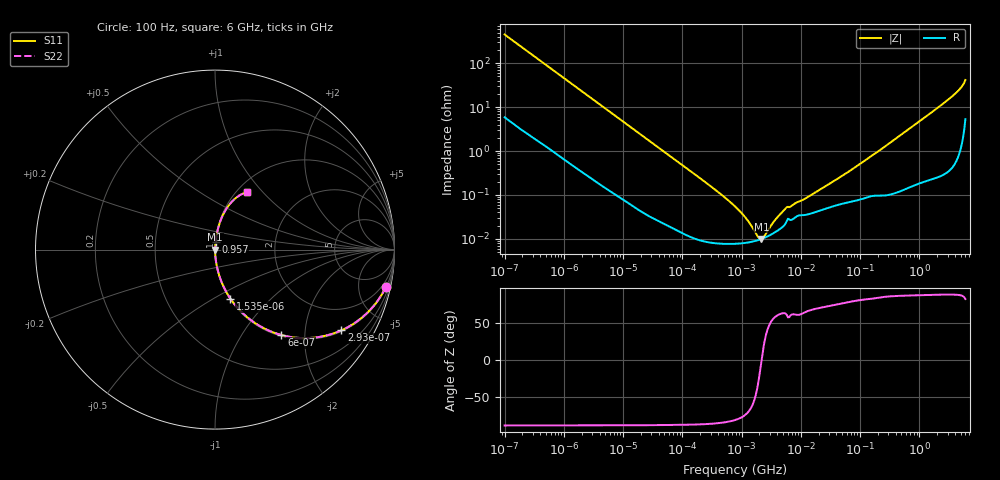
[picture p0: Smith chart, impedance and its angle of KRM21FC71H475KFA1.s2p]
!Murata Part Number: KRM21FC71H475KFA1
!These Parameters are Measured in Series Mode Connection
!Data Generated on Jan 08, 2026
!  o--ll--o
!Port1  Port2
!  o------o
!Operation Temp=25[degC], DC Bias Voltage=0[V]
!Freq. Start=100[Hz] Stop=6[GHz] 401[Steps]
# Hz S RI R 50
!Freq.(Hz) S11(Real) S11(Imag) S21(Real) S21(Imag) S12(Real) S12(Imag) S22(Real) S22(Imag)
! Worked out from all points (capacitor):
!   401 points, 100 Hz to 6 GHz, reference 50 ohm
!   read as one part in series: C = 3.52 uF near 109 Hz
!   lowest |Z| = 9.97 mohm at 2.169 MHz (marker M1)
!   series resonance near 2.178 MHz, so ESL is about 1.5 nH
!   S11 on the Smith chart (normalised r, x): 100 Hz: 1.12, -9.02; 293 Hz: 1.04, -3.11; 600 Hz: 1.02, -1.53; 1.535 kHz: 1.01, -0.60; 957 MHz: 1.00, +0.09; 6 GHz: 1.11, +0.82
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100  0.9507 -0.2102  0.0493 0.2102  0.0493 0.2102  0.9507 -0.2102
179  0.8619 -0.3386  0.1381 0.3386  0.1381 0.3386  0.8619 -0.3386
293  0.7046 -0.4496  0.2954 0.4496  0.2954 0.4496  0.7046 -0.4496
600  0.3702 -0.4759  0.6298 0.4759  0.6298 0.4759  0.3702 -0.4759
938  0.1971 -0.3908  0.8029 0.3908  0.8029 0.3908  0.1971 -0.3908
1535  0.0862 -0.2737  0.9138 0.2737  0.9138 0.2737  0.0862 -0.2737
2008  0.0533 -0.2175  0.9467 0.2175  0.9467 0.2175  0.0533 -0.2175
6728  0.00591 -0.0691  0.9941 0.0691  0.9941 0.0691  0.00591 -0.0691
40335  0.000391 -0.0118  0.9996 0.0118  0.9996 0.0118  0.000391 -0.0118
302498  8.45e-05 -0.00157  0.9999 0.00157  0.9999 0.00157  8.45e-05 -0.00157
774597  7.77e-05 -0.000545  0.9999 0.000545  0.9999 0.000545  7.77e-05 -0.000545
1212075  8.19e-05 -0.000274  0.9999 0.000274  0.9999 0.000274  8.19e-05 -0.000274
1896632  9.37e-05 -6.04e-05  0.9999 6.04e-05  0.9999 6.04e-05  9.37e-05 -6.04e-05
2169299  9.97e-05 -1.6e-06  0.9999 1.6e-06  0.9999 1.6e-06  9.97e-05 -1.6e-06
2481164  0.000107 5.63e-05  0.9999 -5.63e-05  0.9999 -5.63e-05  0.000107 5.63e-05
3712478  0.000143 0.000233  0.9999 -0.000233  0.9999 -0.000233  0.000143 0.000233
5554849  0.000227 0.000441  0.9998 -0.000441  0.9998 -0.000441  0.000227 0.000441
1.555665e7  0.000386 0.000959  0.9996 -0.000959  0.9996 -0.000959  0.000386 0.000959
3.124326e8  0.00123 0.015  0.9988 -0.015  0.9988 -0.015  0.00123 0.015
9.569533e8  0.00381 0.045  0.9962 -0.045  0.9962 -0.045  0.00381 0.045
3.666503e9  0.0356 0.1736  0.9644 -0.1736  0.9644 -0.1736  0.0356 0.1736
6e9  0.1766 0.3223  0.8234 -0.3223  0.8234 -0.3223  0.1766 0.3223
